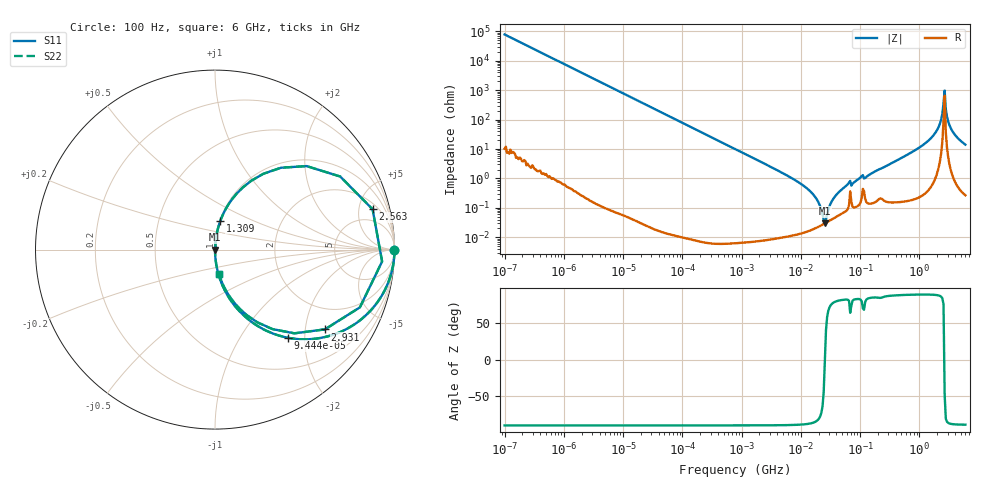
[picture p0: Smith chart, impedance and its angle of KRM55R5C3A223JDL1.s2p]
!Murata Part Number: KRM55R5C3A223JDL1
!These Parameters are Measured in Series Mode Connection
!Data Generated on Jan 08, 2026
!  o--ll--o
!Port1  Port2
!  o------o
!Operation Temp=25[degC], DC Bias Voltage=0[V]
!Freq. Start=100[Hz] Stop=6[GHz] 401[Steps]
# Hz S RI R 50
!Freq.(Hz) S11(Real) S11(Imag) S21(Real) S21(Imag) S12(Real) S12(Imag) S22(Real) S22(Imag)
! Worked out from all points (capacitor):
!   401 points, 100 Hz to 6 GHz, reference 50 ohm
!   read as one part in series: C = 20.3 nF near 109 Hz
!   lowest |Z| = 29.7 mohm at 25.46 MHz (marker M1)
!   series resonance near 25.47 MHz, so ESL is about 1.9 nH
!   S11 on the Smith chart (normalised r, x): 100 Hz: open; 94.44 kHz: 1.00, -1.66; 1.309 GHz: 1.01, +0.33; 2.563 GHz: 2.73, +6.88; 2.931 GHz: 1.23, -2.55; 6 GHz: 1.01, -0.28
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100  1 -0.00128  1.8e-06 0.00128  1.8e-06 0.00128  1 -0.00128
2008  0.9993 -0.0256  0.00066 0.0256  0.00066 0.0256  0.9993 -0.0256
15062  0.9643 -0.1856  0.0357 0.1856  0.0357 0.1856  0.9643 -0.1856
40335  0.7902 -0.4071  0.2098 0.4071  0.2098 0.4071  0.7902 -0.4071
94437  0.4073 -0.4913  0.5927 0.4913  0.5927 0.4913  0.4073 -0.4913
231233  0.1029 -0.3037  0.8971 0.3037  0.8971 0.3037  0.1029 -0.3037
774597  0.0101 -0.0999  0.9899 0.0999  0.9899 0.0999  0.0101 -0.0999
6948629  0.00022 -0.0104  0.9998 0.0104  0.9998 0.0104  0.00022 -0.0104
1.555665e7  0.000191 -0.00312  0.9998 0.00312  0.9998 0.00312  0.000191 -0.00312
1.946e7  0.000226 -0.00165  0.9998 0.00165  0.9998 0.00165  0.000226 -0.00165
2.545746e7  0.000297 -2.7e-06  0.9997 2.7e-06  0.9997 2.7e-06  0.000297 -2.7e-06
3.64232e7  0.000454 0.00218  0.9995 -0.00218  0.9995 -0.00218  0.000454 0.00218
6.233367e7  0.000962 0.00634  0.999 -0.00634  0.999 -0.00634  0.000962 0.00634
3.124326e8  0.00244 0.03  0.9976 -0.03  0.9976 -0.03  0.00244 0.03
1.309207e9  0.0301 0.1612  0.9699 -0.1612  0.9699 -0.1612  0.0301 0.1612
1.95892e9  0.1546 0.346  0.8454 -0.346  0.8454 -0.346  0.1546 0.346
2.34314e9  0.5103 0.4653  0.4897 -0.4653  0.4897 -0.4653  0.5103 0.4653
2.562649e9  0.8781 0.2248  0.1219 -0.2248  0.1219 -0.2248  0.8781 0.2248
2.931063e9  0.6121 -0.4446  0.3879 0.4446  0.3879 0.4446  0.6121 -0.4446
3.205649e9  0.32 -0.4429  0.68 0.4429  0.68 0.4429  0.32 -0.4429
3.666503e9  0.1391 -0.3312  0.8609 0.3312  0.8609 0.3312  0.1391 -0.3312
6e9  0.0221 -0.1377  0.9779 0.1377  0.9779 0.1377  0.0221 -0.1377
